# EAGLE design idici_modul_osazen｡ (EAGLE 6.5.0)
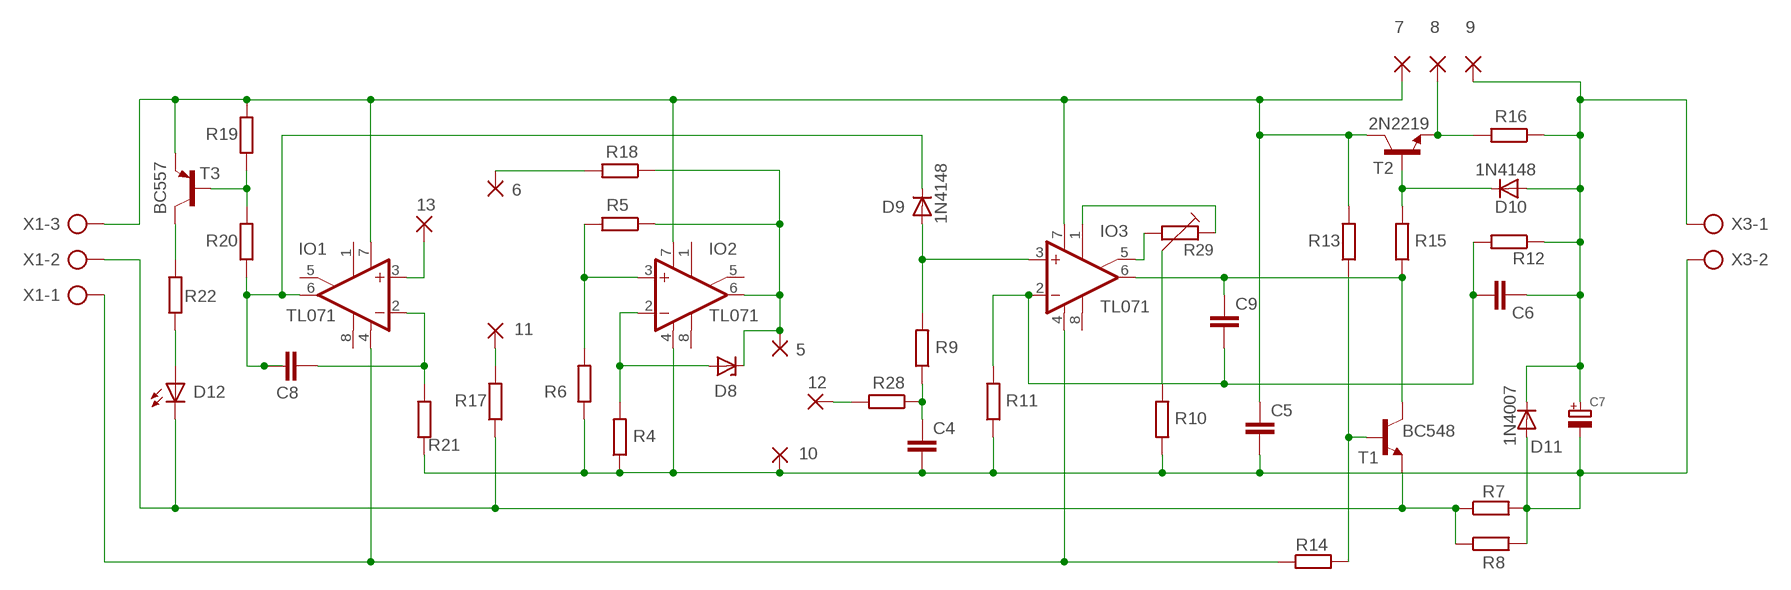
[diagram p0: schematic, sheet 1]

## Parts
5  WIREPAD2,54/1,0  [2,54/1,0]
6  WIREPAD2,54/1,0  [2,54/1,0]
7  WIREPAD2,54/1,0  [2,54/1,0]
8  WIREPAD2,54/1,0  [2,54/1,0]
9  WIREPAD2,54/1,0  [2,54/1,0]
10  WIREPAD2,54/1,0  [2,54/1,0]
11  WIREPAD2,54/1,0  [2,54/1,0]
12  WIREPAD2,54/1,0  [2,54/1,0]
13  WIREPAD2,54/1,0  [2,54/1,0]
C4  CK  [C3X5]
C5  WIMA-RM5-3,5  [C5-3,5X7]
C6  CK  [C3X5]
C7  ELETKROLYT-5X10-RAD  [ELYT-5RM_10MM/RAD]
C8  CK  [C3X5]
C9  CK  [C3X5]
D8  BZX85  [DO41Z10]
D9  1N4148  [DO35-10]
D10  1N4148  [DO35-10]
D11  1N4007  [DO41-10]
D12  LED5MM  [LED5MM]
IO1  TL071  TL071P  [DIL08]
IO2  TL071  TL071P  [DIL08]
IO3  TL071  TL071P  [DIL08]
R4  R-EU_0207/7  [0207/7]
R5  R-EU_0207/7  [0207/7]
R6  R-EU_0207/7  [0207/7]
R7  R-EU_0922/22  [0922/22]
R8  R-EU_0922/22  [0922/22]
R9  R-EU_0207/7  [0207/7]
R10  R-EU_0207/7  [0207/7]
R11  R-EU_0207/7  [0207/7]
R12  R-EU_0207/7  [0207/7]
R13  R-EU_0207/7  [0207/7]
R14  R-EU_0207/7  [0207/7]
R15  R-EU_0207/7  [0207/7]
R16  R-EU_0207/7  [0207/7]
R17  R-EU_0207/7  [0207/7]
R18  R-EU_0207/7  [0207/7]
R19  R-EU_0207/7  [0207/7]
R20  R-EU_0207/7  [0207/7]
R21  R-EU_0207/7  [0207/7]
R22  R-EU_0207/7  [0207/7]
R28  R-EU_0207/7  [0207/7]
R29  PT-6_V-LEZ  [PT6V]
T1  BC548  [TO92-EBC]
T2  2N2219  [TO5]
T3  BC557  [TO92]
X1  AK500/3-H  [AK500/3-H]
X3  AK500/2-H  [AK500/2-H]

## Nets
N$1: 7.1(P) C5.1 IO1.7(V+) IO2.7(V+) IO3.7(V+) R13.2 R19.2 T2.3(C) T3.1(E) X1.3
N$2: R22.2 T3.3(C)
N$3: D12.A R22.1
N$4: IO3.5(ON2) R29.2
N$5: IO1.4(V-) IO3.4(V-) R14.1 X1.1
N$6: R19.1 R20.2 T3.2(B)
N$7: C8.1 D9.C IO1.6(OUT) R20.1
N$8: C8.2 IO1.2(-IN) R21.2
N$9: 13.1(P) IO1.3(+IN)
N$10: 11.1(P) R17.2
N$11: 12.1(P) R28.2
N$12: D8.A IO2.2(-IN) R4.2
N$13: IO2.3(+IN) R5.2 R6.2
N$14: 6.1(P) R18.2
N$15: 5.1(P) D8.C IO2.6(OUT) R5.1 R18.1
N$16: R10.2 R29.3
N$18: C4.1 R9.1 R28.1
N$19: D9.A IO3.3(+IN) R9.2
N$20: C6.1 C9.2 IO3.2(-IN) R11.2 R12.2
N$21: IO3.1(ON1) R29.1
N$22: C9.1 IO3.6(OUT) R15.1 T1.C
N$23: 8.1(P) R16.2 T2.1(E)
N$24: R13.1 R14.2 T1.B
N$25: 9.1(P) C6.2 C7.P$1(+) D10.A D11.C R12.1 R16.1 X3.1
N$26: D10.C R15.2 T2.2(B)
N$27: 10.1(P) C4.2 C5.2 C7.P$2(-) D11.A IO2.4(V-) R4.1 R6.1 R7.2 R8.2 R10.1 R11.1 R21.1 X3.2
N$28: D12.K(C) R7.1 R8.1 R17.1 T1.E X1.2
Unconnected: IO1.1(ON1) IO1.5(ON2) IO1.8(OPT) IO2.1(ON1) IO2.5(ON2) IO2.8(OPT) IO3.8(OPT)

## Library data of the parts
5-13 = wirepad:WIREPAD: Wire PAD connect wire on PCB
C4 C6 C8 C9 = kondenzatory:CK: Keramické kondenzátory rady CK
C5 = kondenzatory:WIMA-RM5: Kondenzátory fóliové WIMA RM 5
C7 = Kondenzátory:ELETKROLYT: ELEKTROLYTICKÝ KONDENZÁTOR
D8 = diode:BZX85: Z DIODE
D9 D10 = diody:1N4148: Univerzální dioda
D11 = diody:1N4007: Usmernovací dioda
D12 = led:LED: LED
IO1-IO3 = linear:TL071: OP AMP
R4-R22 R28 = resistor:R-EU_: RESISTOR, European symbol
R29 = #PaJa_21:PT-6: Trimr PT6 - 6,3mm
T1 = transistor-npn:BC548*: NPN Transistor
T2 = tranzistory NPN:2N2219: NPN TRANSISTOR
T3 = transistor-pnp:BC557: PNP Transistor
X1 = con-ptr500:AK500/3-H: CONNECTOR Aug. 2004 / PTR Meßtechnik: Die Bezeichnung der Serie AK505 wurde geändert. Es handelt sich hierbei um AK500 in horizontaler Ausführung.; OC_FARNELL: unknown; OC_NEWARK: unknown
X3 = con-ptr500:AK500/2-H: CONNECTOR; OC_FARNELL: unknown; OC_NEWARK: unknown

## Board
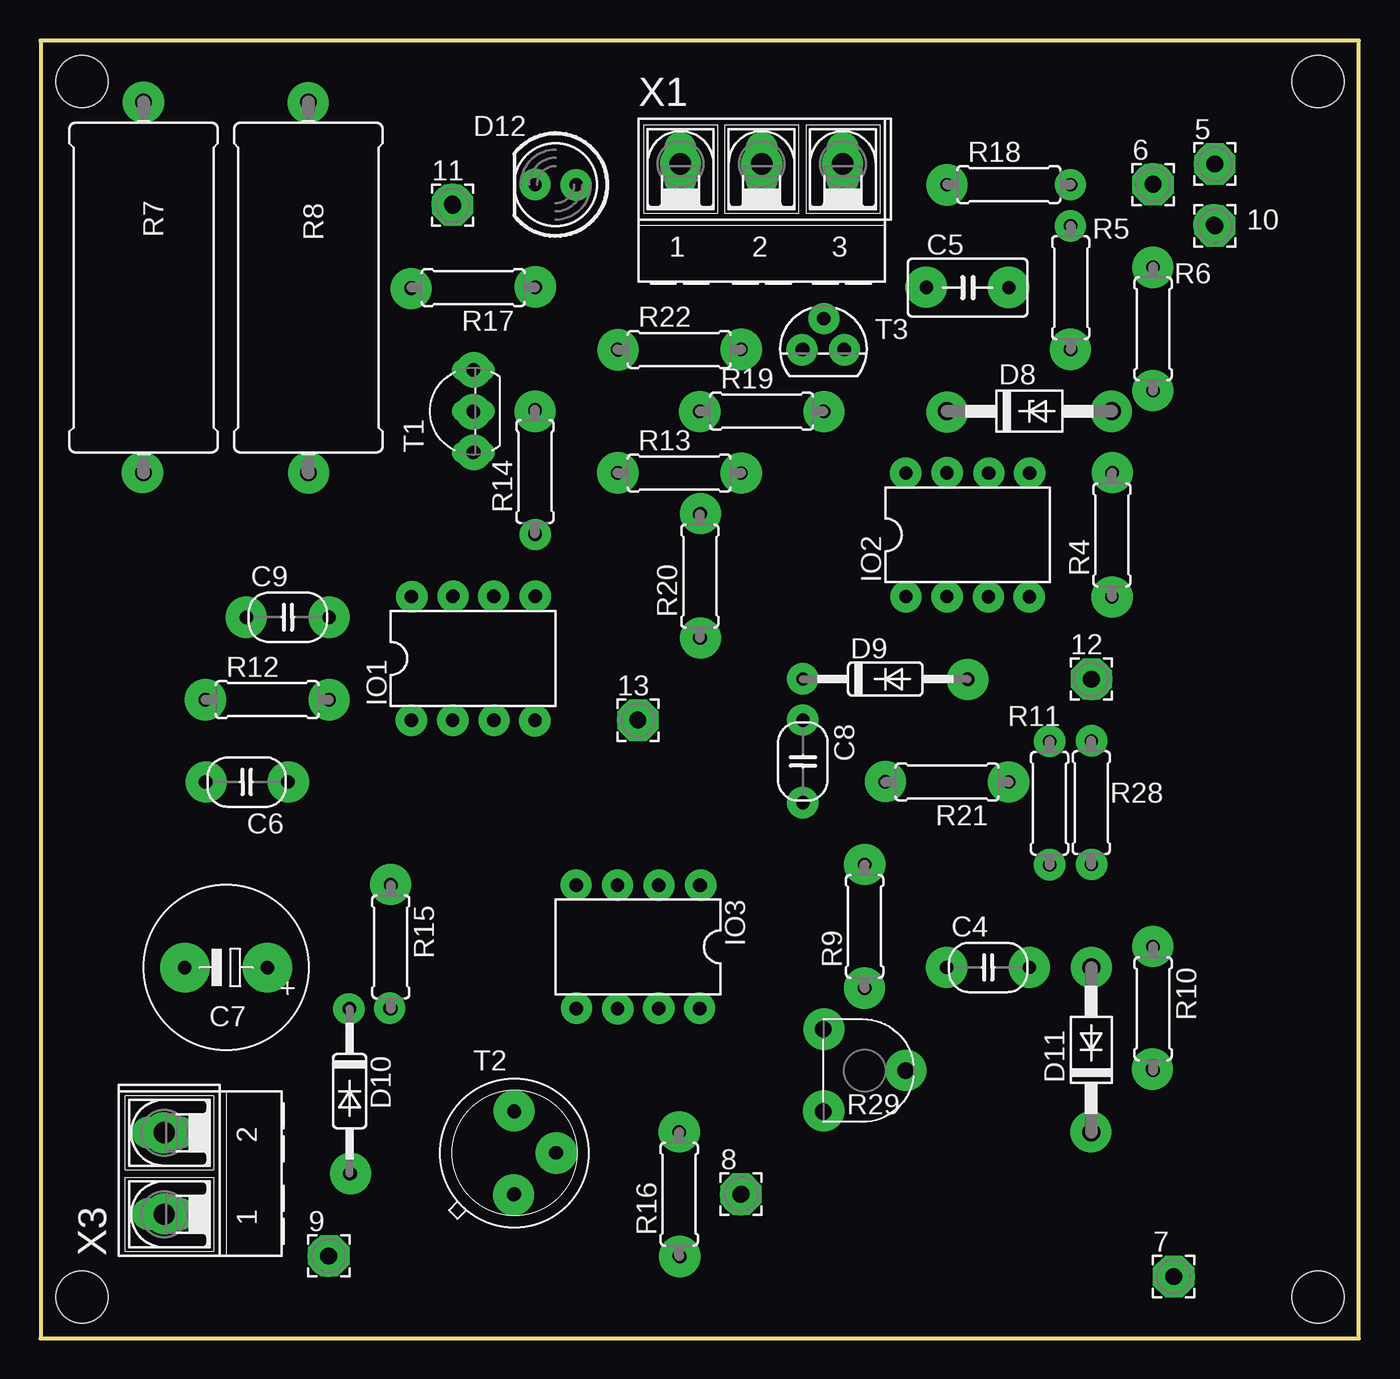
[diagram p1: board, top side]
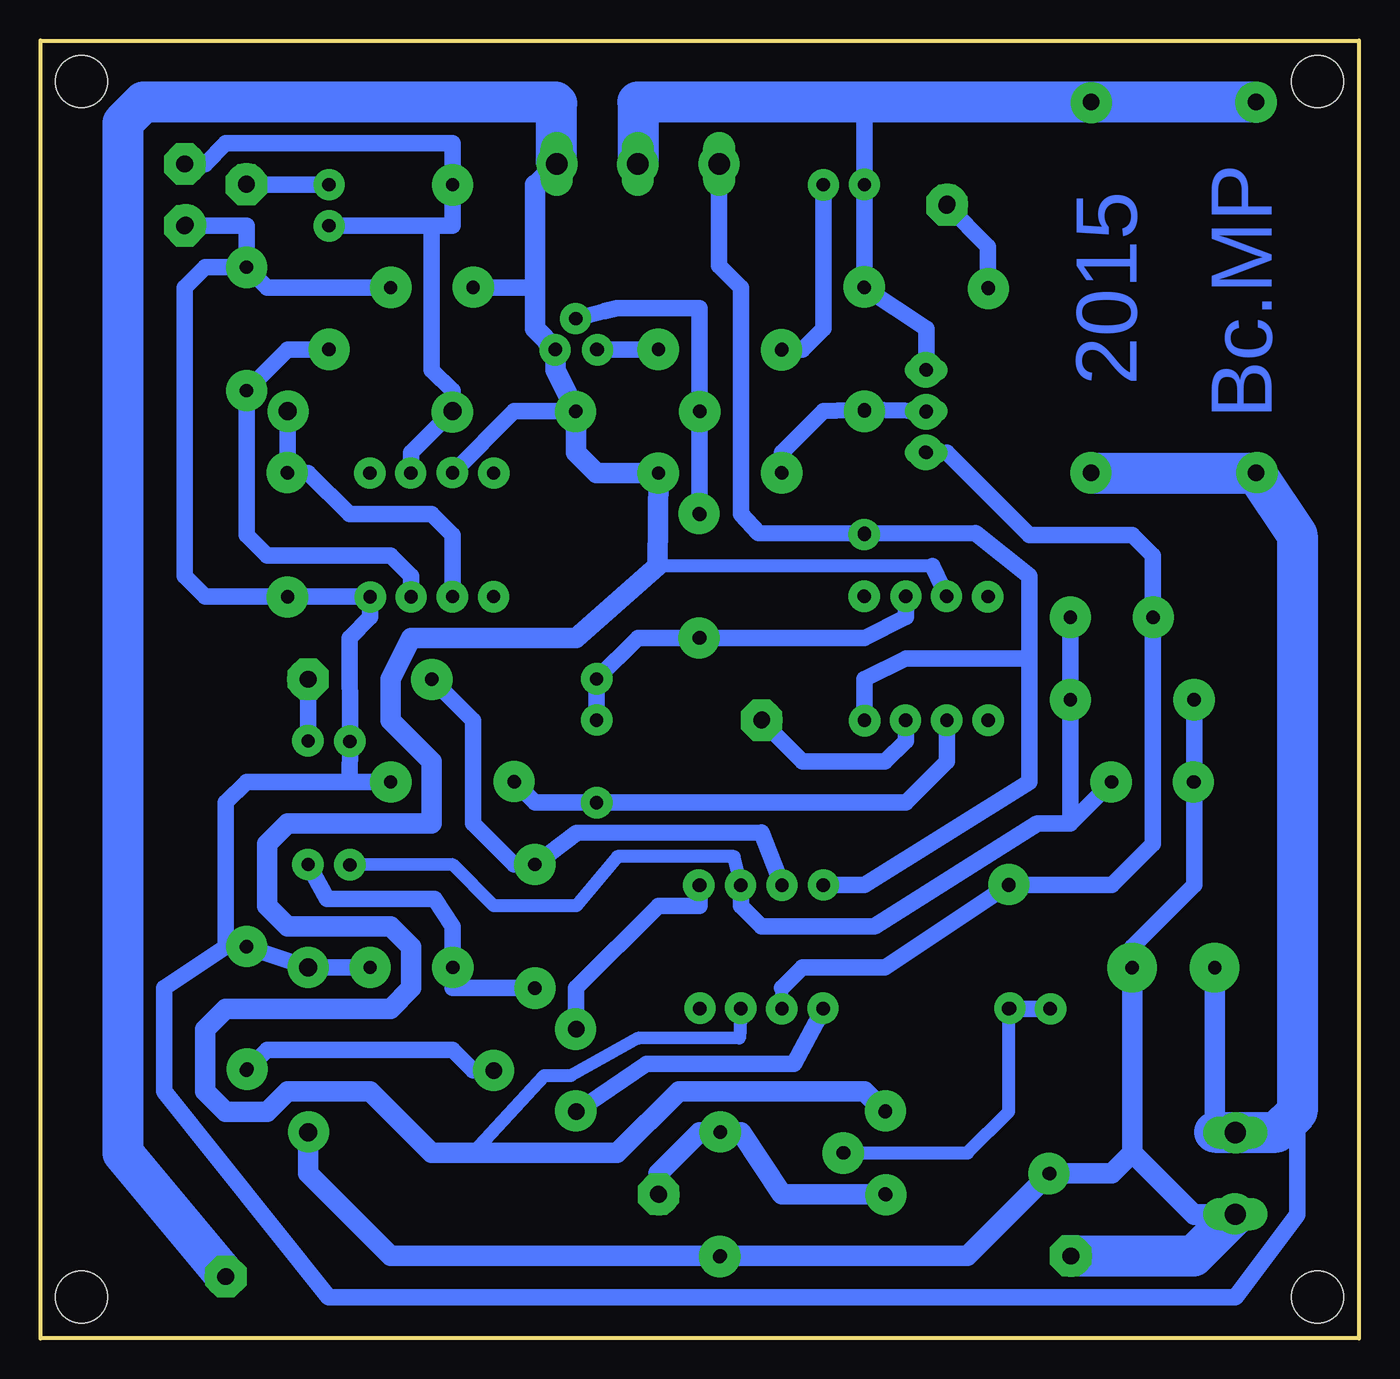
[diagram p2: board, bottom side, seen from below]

Size 81.27 x 80 mm. Coordinates in mm from the lower left corner, seen from the top.
Outline: 0,0 81.27,0 81.27,80 0,80 0,0
Copper layers (1*16): Top 0.035mm / dielectric 1.5mm / Bottom 0.035mm
Design rules "default": minimum track width 10mil, minimum drill 24mil, track to track 8mil, track to pad 8mil, pad to pad 8mil, via to via 8mil, smd to smd 8mil, copper to edge 40mil, drill to drill 8mil, minimum pad ring 10mil, minimum via ring 8mil, stop-mask expansion 4mil, vias tented up to drill 0mil, thermal gap 10mil
Holes 3.2 mm at 2.54,77.47 78.74,77.47 78.74,2.54 2.54,2.54

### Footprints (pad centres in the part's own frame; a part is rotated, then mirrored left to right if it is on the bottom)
2,54/1,0 = drill 1.016 pad 2.54 octagon: 1 0,0
C3X5 = drill 0.813 pad 1.422 octagon: 1 -2.54,0; 2 2.54,0
C5-3,5X7 = drill 0.813 pad 1.6 octagon: 1 -2.54,0; 2 2.54,0
ELYT-5RM_10MM/RAD = drill 0.8 pad 3.048: P$1 -2.54,0; P$2 2.54,0
DO41Z10 = drill 1.118: A 5.08,0; C -5.08,0
DO35-10 = drill 0.813 pad 1.676 octagon: A 5.08,0 | drill 0.813 pad 1.676: C -5.08,0
DO41-10 = drill 1.118 pad 1.778 octagon: A 5.08,0 | drill 1.118 pad 1.778: C -5.08,0
LED5MM = drill 0.813 octagon: A -1.27,0; K 1.27,0
DIL08 = drill 0.813 pad 1.27: 1 -3.81,-3.81; 2 -1.27,-3.81; 3 1.27,-3.81; 4 3.81,-3.81; 5 3.81,3.81; 6 1.27,3.81; 7 -1.27,3.81; 8 -3.81,3.81
0207/7 = drill 0.813 octagon: 1 -3.81,0; 2 3.81,0
0922/22 = drill 1.016 octagon: 1 -11.43,0; 2 11.43,0
PT6V = drill 1.016 pad 2.184 octagon: 1 -2.54,-2.54; 2 2.54,-2.54; 3 0,2.54
TO92-EBC = drill 0.813 long: B 0,-1.27; C -2.54,-1.27; E 2.54,-1.27
TO5 = drill 0.813 octagon: 1 0,-2.54; 2 2.54,0; 3 0,2.54
TO92 = drill 0.813 octagon: 1 1.27,0; 2 0,1.905; 3 -1.27,0
AK500/3-H = drill 1.321 long: 1 -5.004,0; 2 0,0; 3 5.004,0
AK500/2-H = drill 1.321 long: 1 -2.515,0; 2 2.515,0

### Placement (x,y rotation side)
5  72.39,72.39 0 top
6  68.58,71.12 0 top
7  69.85,3.81 0 top
8  43.18,8.89 0 top
9  17.78,5.08 0 top
10  72.39,68.58 0 top
11  25.4,69.85 0 top
12  64.77,40.64 0 top
13  36.83,38.1 0 top
C4  58.42,22.86 0 top
C5  57.15,64.77 0 top
C6  12.7,34.29 180 top
C7  11.43,22.86 180 top
C8  46.99,35.56 270 top
C9  15.24,44.45 0 top
D8  60.96,57.15 0 top
D9  52.07,40.64 0 top
D10  19.05,15.24 270 top
D11  64.77,17.78 90 top
D12  31.75,71.12 180 top
IO1  26.67,41.91 0 top
IO2  57.15,49.53 0 top
IO3  36.83,24.13 180 top
R4  66.04,49.53 90 top
R5  63.5,64.77 270 top
R6  68.58,62.23 270 top
R7  6.35,64.77 270 top
R8  16.51,64.77 270 top
R9  50.8,25.4 90 top
R10  68.58,20.32 270 top
R11  62.2,32.99 270 top
R12  13.97,39.37 0 top
R13  39.37,53.34 0 top
R14  30.48,53.43 90 top
R15  21.59,24.13 270 top
R16  39.37,8.89 90 top
R17  26.67,64.77 180 top
R18  59.69,71.12 0 top
R19  44.45,57.15 0 top
R20  40.64,46.99 90 top
R21  55.88,34.29 180 top
R22  39.37,60.96 0 top
R28  64.77,33.02 90 top
R29  50.8,16.51 270 top
T1  25.4,57.15 90 top
T2  29.21,11.43 0 top
T3  48.26,60.96 0 top
X1  44.45,72.39 0 top
X3  7.62,10.16 90 top

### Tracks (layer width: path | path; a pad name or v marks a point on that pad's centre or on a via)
N$1
  Bottom 0.406: 49.45,76.12 49.53,76.2
  Bottom 0.813: IO3.7 38.2,18.5 44.4,18.51 48.59,16.18 50.23,16.18 54.61,11.43 | 26.3,47.61 29.06,47.61 43.24,47.61
  Bottom 1.016: IO1.7 26.3,47.61 | IO2.7 52.07,57.15 R19.2 | 50.8,71.12 50.72,71.12 | C5.1 50.8,64.77
  Bottom 1.27: 50.8,71.12 50.8,64.77 50.8,62.23 T3.1 49.53,59.69 R19.2 48.26,54.61 46.99,53.34 R13.2 43.24,47.61 48.26,43.18 58.42,43.18 59.69,40.64 59.69,38.1 57.15,35.56 57.15,31.75 66.04,31.75 67.31,30.48 67.31,26.67 66.04,25.4 59.69,25.4 58.42,24.13 58.42,21.59 59.69,20.32 69.85,20.32 71.12,19.05 71.12,15.24 69.85,13.97 67.31,13.97 66.04,15.24 60.96,15.24 57.15,11.43 54.61,11.43 45.72,11.43 41.91,15.24 30.48,15.24 T2.3 | 50.72,71.12 X1.3
  Bottom 2.54: 7.1 76.2,11.43 76.2,74.93 74.93,76.2 49.53,76.2 | X1.3 49.45,76.12
N$2
  Bottom 1.016: R22.2 T3.3
N$3
  Bottom 1.016: R22.1 34.29,60.96 33.02,62.23 D12.A
N$4
  Bottom 1.016: IO3.5 34.82,16.92 43.92,16.92 R29.2
N$5
  Bottom 1.016: IO3.4 30.48,27.94 20.32,34.29 20.32,41.91 | X1.1 39.45,66.12 38.1,64.77 38.1,50.8 37.02,49.63 R14.1 23.64,49.63 20.32,46.99 20.32,41.91 | IO1.4 30.48,40.64 27.94,41.91 20.32,41.91
N$6
  Bottom 1.016: R20.2 R19.1 40.64,63.5 45.72,63.5 46.52,63.32 T3.2
N$7
  Bottom 1.016: C8.1 D9.C 44.45,43.18 R20.1 30.48,43.18 27.94,44.45 IO1.6
N$8
  Bottom 1.016: IO1.2 25.4,35.56 27.94,33.02 C8.2 50.8,33.02 R21.2
N$9
  Bottom 1.016: IO1.3 27.94,36.83 29.21,35.56 34.29,35.56 13.1
N$10
  Bottom 1.016: R17.2 22.86,67.31 11.1
N$11
  Bottom 1.016: R28.2 12.1
N$12
  Bottom 1.016: D8.A R4.2 64.77,53.34 62.23,50.8 57.15,50.8 55.88,49.53 IO2.2
N$13
  Bottom 1.016: R5.2 66.04,60.96 R6.2 68.58,49.53 67.31,48.26 59.69,48.26 58.42,46.99 IO2.3
N$14
  Bottom 1.016: R18.2 6.1
N$15
  Bottom 1.016: 5.1 71.12,72.39 69.85,73.66 55.88,73.66 R18.1 55.88,68.58 57.15,68.58 | R5.1 57.15,68.58 | IO2.6 58.42,54.61 D8.C 55.88,58.42 57.15,59.69 57.15,68.58
N$16
  Bottom 1.016: R29.3 54.61,16.51 55.88,17.78 67.31,17.78 R10.2
N$17  (via drill 0.8 pad 2.54)
  other vias: 6.35,76.2
N$18
  Bottom 1.016: R9.1 55.88,21.59 C4.1 55.88,25.4 56.99,27.09 63.6,27.09 R28.1
N$19
  Bottom 1.016: IO3.3 36.82,31.2 48.22,31.16 R9.2 52.07,29.21 54.61,31.75 54.61,38.1 D9.A
N$20
  Bottom 0.813: IO3.2 38.51,29.7 45.71,29.7 48.26,26.67 53.34,26.67 55.88,29.21 R11.2
  Bottom 1.016: 17.78,31.75 R12.2 C9.2 | C6.1 17.78,31.75 | IO3.2 38.1,26.67 36.83,25.4 29.86,25.4 19.83,31.75 17.78,31.75
N$21
  Bottom 1.016: IO3.1 40.64,26.67 43.18,26.67 48.26,21.59 R29.1
N$22
  Bottom 0.406: 25.4,54.61 T1.C
  Bottom 0.813: IO3.6 35.56,21.59
  Bottom 1.016: 35.56,21.59 34.29,22.86 29.21,22.86 R15.1 15.24,27.94 12.7,30.48 C9.1 12.7,48.26 13.97,49.53 20.32,49.53 25.4,54.61
N$23
  Bottom 1.27: T2.1 35.56,8.89 38.1,12.7 R16.2 40.64,12.7 43.18,10.16 8.1
N$24
  Bottom 1.016: T1.B R14.2 33.02,57.15 35.56,54.61 R13.1
N$25
  Bottom 0.406: C7.P$1 13.97,24.13
  Bottom 0.813: 10.13,7.64 10.16,7.62
  Bottom 1.016: R12.1 C6.2 10.16,27.94 13.97,24.13 | 64.77,11.43 D11.C
  Bottom 1.27: 13.97,11.43 C7.P$1 | 13.97,11.43 15.24,10.16 D10.A 24.13,5.08 R16.1 59.69,5.08 64.77,10.16 D11.C | X3.1 10.13,7.64 | 10.16,7.62 13.97,11.43
  Bottom 2.54: 9.1 10.19,5.08 X3.1
N$26
  Bottom 0.813: T2.2 24.13,11.43 21.59,13.97 R15.2
  Bottom 1.016: R15.2 D10.C
N$27
  Bottom 0.406: X3.2 8.87,12.68 8.89,12.7
  Bottom 1.016: C4.2 D11.A R10.1 69.85,24.13 | C5.2 67.31,64.77 R6.1 | 10.1 68.58,68.58 R6.1 | X3.2 3.81,13.97 3.81,7.62 7.62,2.54 63.5,2.54 73.66,15.24 73.66,21.59 69.85,24.13 | R6.1 71.12,66.04 72.39,64.77 72.39,46.99 71.12,45.72 R4.1 IO2.4 60.96,44.45 62.23,43.18 R11.1 62.23,34.29 | R21.1 62.23,34.29 | 62.23,34.29 68.58,34.29 69.85,33.02 69.85,24.13
  Bottom 1.27: C7.P$2 8.89,12.7
  Bottom 2.54: R8.2 R7.2 3.81,49.53 3.81,13.97 5.08,12.7 8.89,12.7
N$28
  Bottom 1.016: T1.E 26.67,62.23 R17.1 D12.K 30.48,76.2
  Bottom 2.54: R7.1 R8.1 30.48,76.2 44.45,76.2 X1.2
N$29  (via drill 0.8 pad 2.54)
  other vias: 16.5,76.17
N$30  (via drill 1 pad 2.54)
  other vias: 25.39,69.92
N$31  (via drill 1 pad 2.54)
  other vias: 39.45,72.4
N$32  (via drill 1 pad 2.54)
  other vias: 44.46,72.36
N$33  (via drill 1 pad 2.54)
  other vias: 49.44,72.4
N$34  (via drill 1 pad 2.54)
  other vias: 72.38,72.4
N$35  (via drill 1 pad 2.54)
  other vias: 72.33,68.65
N$36  (via drill 1 pad 2.54)
  other vias: 68.58,71.18
N$37  (via drill 1 pad 2.54)
  other vias: 64.8,40.63
N$38  (via drill 1 pad 2.54)
  other vias: 36.79,38.13
N$39  (via drill 1 pad 2.54)
  other vias: 17.73,5.08
N$40  (via drill 1 pad 2.54)
  other vias: 43.15,8.87
N$41  (via drill 1 pad 2.54)
  other vias: 69.87,3.8
N$42  (via drill 1 pad 2.54)
  other vias: 7.65,7.67
N$43  (via drill 1 pad 2.54)
  other vias: 7.59,12.66
N$44  (via drill 0.8 pad 2.54)
  other vias: 16.53,53.35
N$45  (via drill 0.8 pad 2.54)
  other vias: 6.28,53.36
N$46  (via drill 0.8 pad 2.54)
  other vias: 22.84,64.71
N$47  (via drill 0.8 pad 2.54)
  other vias: 30.5,64.81
N$48  (via drill 0.8 pad 2.54)
  other vias: 35.6,60.93
N$49  (via drill 0.8 pad 2.18)
  other vias: 26.71,59.71
N$50  (via drill 0.8 pad 2.18)
  other vias: 26.68,57.11
N$51  (via drill 0.8 pad 2.18)
  other vias: 26.72,54.62
N$52  (via drill 0.8 pad 1.93)
  other vias: 48.29,62.86
N$53  (via drill 0.8 pad 1.93)
  other vias: 49.56,60.94
N$54  (via drill 0.8 pad 1.93)
  other vias: 46.93,60.94
N$55  (via drill 0.8 pad 1.93)
  other vias: 33.01,71.1
N$56  (via drill 0.8 pad 1.93)
  other vias: 30.48,71.13
N$57  (via drill 0.8 pad 2.54)
  other vias: 55.87,71.1
N$58  (via drill 0.8 pad 1.93)
  other vias: 63.48,71.12
N$59  (via drill 0.8 pad 1.93)
  other vias: 63.48,68.58
N$60  (via drill 0.8 pad 2.54)
  other vias: 68.56,66.02
N$61  (via drill 0.8 pad 2.54)
  other vias: 59.68,64.78
N$62  (via drill 0.8 pad 2.54)
  other vias: 63.48,60.96
N$63  (via drill 0.8 pad 2.54)
  other vias: 68.56,58.43
N$64  (via drill 0.8 pad 2.54)
  other vias: 66.01,57.14
N$65  (via drill 0.8 pad 2.54)
  other vias: 55.88,57.1
N$66  (via drill 0.8 pad 2.54)
  other vias: 54.6,64.8
N$67  (via drill 0.8 pad 2.54)
  other vias: 48.29,57.12
N$68  (via drill 0.8 pad 2.54)
  other vias: 43.19,60.96
N$69  (via drill 0.8 pad 2.54)
  other vias: 40.63,57.12
N$70  (via drill 0.8 pad 2.54)
  other vias: 43.19,53.34
N$71  (via drill 0.8 pad 2.54)
  other vias: 35.59,53.36
N$72  (via drill 0.8 pad 2.54)
  other vias: 30.48,57.14
N$73  (via drill 0.8 pad 2.54)
  other vias: 66.08,53.37
N$74  (via drill 0.8 pad 2.54)
  other vias: 66.05,45.69
N$75  (via drill 0.8 pad 1.93)
  other vias: 60.98,53.34
N$76  (via drill 0.8 pad 1.93)
  other vias: 58.46,53.34
N$77  (via drill 0.8 pad 1.93)
  other vias: 55.88,53.37
N$78  (via drill 0.8 pad 1.93)
  other vias: 53.33,53.34
N$79  (via drill 0.8 pad 1.93)
  other vias: 53.34,45.71
N$80  (via drill 0.8 pad 1.93)
  other vias: 55.88,45.71
N$81  (via drill 0.8 pad 1.93)
  other vias: 58.42,45.7
N$82  (via drill 0.8 pad 1.93)
  other vias: 60.95,45.7
N$83  (via drill 0.8 pad 1.93)
  other vias: 33.01,27.95
N$84  (via drill 0.8 pad 1.93)
  other vias: 35.57,27.93
N$85  (via drill 0.8 pad 1.93)
  other vias: 38.12,27.93
N$86  (via drill 0.8 pad 1.93)
  other vias: 40.69,27.93
N$87  (via drill 0.8 pad 1.93)
  other vias: 40.62,20.35
N$88  (via drill 0.8 pad 1.93)
  other vias: 38.12,20.35
N$89  (via drill 0.8 pad 1.93)
  other vias: 35.58,20.31
N$90  (via drill 0.8 pad 1.93)
  other vias: 33.04,20.35
N$91  (via drill 0.8 pad 1.93)
  other vias: 22.88,45.72
N$92  (via drill 0.8 pad 1.93)
  other vias: 25.43,45.75
N$93  (via drill 0.8 pad 1.93)
  other vias: 27.93,45.75
N$94  (via drill 0.8 pad 1.93)
  other vias: 30.5,45.75
N$95  (via drill 0.8 pad 1.93)
  other vias: 30.48,38.07
N$96  (via drill 0.8 pad 1.93)
  other vias: 27.95,38.1
N$97  (via drill 0.8 pad 1.93)
  other vias: 25.41,38.1
N$98  (via drill 0.8 pad 1.93)
  other vias: 22.86,38.1
N$99  (via drill 0.8 pad 1.93)
  other vias: 30.5,49.54
N$100  (via drill 0.8 pad 2.54)
  other vias: 40.68,50.85
N$101  (via drill 0.8 pad 2.54)
  other vias: 40.68,43.16
N$102  (via drill 0.8 pad 2.54)
  other vias: 12.68,44.44
N$103  (via drill 0.8 pad 2.54)
  other vias: 17.78,44.44
N$104  (via drill 0.8 pad 2.54)
  other vias: 17.79,39.37
N$105  (via drill 0.8 pad 2.54)
  other vias: 10.17,39.37
N$106  (via drill 0.8 pad 2.54)
  other vias: 10.21,34.3
N$107  (via drill 0.8 pad 2.54)
  other vias: 15.28,34.3
N$108  (via drill 0.8 pad 2.54)
  other vias: 21.58,27.97
N$109  (via drill 0.8 pad 1.93)
  other vias: 46.99,33.03
N$110  (via drill 0.8 pad 2.54)
  other vias: 52.09,34.32
N$111  (via drill 0.8 pad 2.54)
  other vias: 50.8,29.21
N$112  (via drill 0.8 pad 2.54)
  other vias: 59.68,34.3
N$113  (via drill 0.8 pad 2.54)
  other vias: 57.16,40.62
N$114  (via drill 0.8 pad 2.54)
  other vias: 68.57,24.16
N$115  (via drill 0.8 pad 2.54)
  other vias: 64.77,22.86
N$116  (via drill 0.8 pad 2.54)
  other vias: 60.95,22.86
N$117  (via drill 0.8 pad 2.54)
  other vias: 55.85,22.86
N$118  (via drill 0.8 pad 2.54)
  other vias: 50.78,21.58
N$119  (via drill 0.8 pad 1.93)
  other vias: 62.21,36.81
N$120  (via drill 0.8 pad 1.93)
  other vias: 64.79,36.83
N$121  (via drill 0.8 pad 1.93)
  other vias: 64.79,29.21
N$122  (via drill 0.8 pad 1.93)
  other vias: 62.21,29.19
N$123  (via drill 0.8 pad 1.93)
  other vias: 46.99,40.65
N$124  (via drill 0.8 pad 1.93)
  other vias: 46.99,38.12
N$125  (via drill 0.8 pad 2.54)
  other vias: 68.54,16.6
N$126  (via drill 0.8 pad 2.54)
  other vias: 64.75,12.73
N$127  (via drill 0.8 pad 2.54)
  other vias: 48.27,14.02
N$128  (via drill 0.8 pad 2.54)
  other vias: 53.35,16.52
N$129  (via drill 0.8 pad 2.54)
  other vias: 39.37,12.73
N$130  (via drill 0.8 pad 2.54)
  other vias: 39.4,5.04
N$131  (via drill 0.8 pad 2.54)
  other vias: 48.29,19.06
N$132  (via drill 0.8 pad 2.54)
  other vias: 19.11,10.16
N$133  (via drill 0.8 pad 2.54)
  other vias: 29.19,14.03
N$134  (via drill 0.8 pad 2.54)
  other vias: 31.8,11.43
N$135  (via drill 0.8 pad 2.54)
  other vias: 29.16,8.85
N$136  (via drill 0.8 pad 1.93)
  other vias: 19.01,20.31
N$137  (via drill 0.8 pad 1.93)
  other vias: 21.51,20.35
N$138  (via drill 0.8 pad 2.54)
  other vias: 8.89,22.83
N$139  (via drill 0.8 pad 2.54)
  other vias: 13.99,22.83

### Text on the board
Bottom: Bc.MP | 2015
